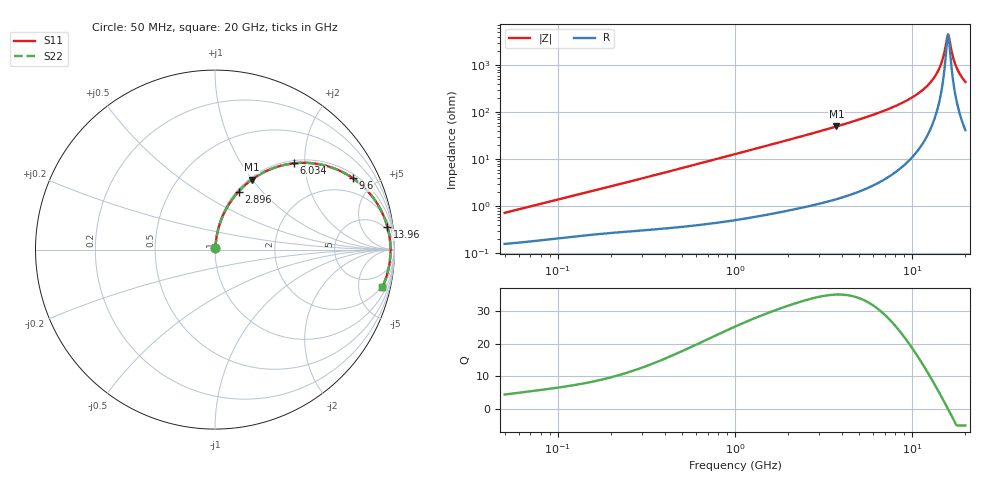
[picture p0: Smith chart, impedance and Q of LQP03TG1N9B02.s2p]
!Murata Part Number: LQP03TG1N9B02
!These Parameters are Measured in Series Mode Connection
!  o--[Z]--o
!Port1  Port2
!  o-------o
!Freq. Start=50[MHz] Stop=20[GHz], 401[Steps]
# Hz S RI R 50
!Freq.(Hz) S11(Real) S11(Imag) S21(Real) S21(Imag) S12(Real) S12(Imag) S22(Real) S22(Imag)
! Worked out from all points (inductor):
!   401 points, 50 MHz to 20 GHz, reference 50 ohm
!   read as one part in series: L = 2.23 nH near 51.52 MHz
!   highest Q = 35.1 at 3.736 GHz (marker M1), where L = 2.11 nH
!   self-resonance near 15.74 GHz
!   S11 on the Smith chart (normalised r, x): 50 MHz: 1.00, +0.01; 2.896 GHz: 1.02, +0.75; 6.034 GHz: 1.06, +1.76; 9.6 GHz: 1.19, +3.74; 13.96 GHz: 3, +14; 20 GHz: 1.83, -8.72
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5e7  0.00163 0.00705  0.9984 -0.00705  0.9984 -0.00705  0.00163 0.00705
1.364002e8  0.0027 0.0183  0.9973 -0.0183  0.9973 -0.0183  0.0027 0.0183
3.721004e8  0.00558 0.0479  0.9944 -0.0479  0.9944 -0.0479  0.00558 0.0479
1e9  0.0209 0.1247  0.9791 -0.1247  0.9791 -0.1247  0.0209 0.1247
2.728004e9  0.1182 0.3084  0.8818 -0.3084  0.8818 -0.3084  0.1182 0.3084
2.896447e9  0.1313 0.3234  0.8687 -0.3234  0.8687 -0.3234  0.1313 0.3234
3.736399e9  0.2039 0.3889  0.7961 -0.3889  0.7961 -0.3889  0.2039 0.3889
6.034176e9  0.4382 0.4807  0.5618 -0.4807  0.5618 -0.4807  0.4382 0.4807
7.442007e9  0.5819 0.4754  0.4181 -0.4754  0.4181 -0.4754  0.5819 0.4754
9.600142e9  0.7673 0.3984  0.2327 -0.3984  0.2327 -0.3984  0.7673 0.3984
1.201863e10  0.9042 0.2554  0.0958 -0.2554  0.0958 -0.2554  0.9042 0.2554
1.314879e10  0.9423 0.1809  0.0577 -0.1809  0.0577 -0.1809  0.9423 0.1809
1.396067e10  0.9605 0.1273  0.0395 -0.1273  0.0395 -0.1273  0.9605 0.1273
1.482269e10  0.9725 0.0715  0.0275 -0.0715  0.0275 -0.0715  0.9725 0.0715
1.573793e10  0.9778 0.0143  0.0222 -0.0143  0.0222 -0.0143  0.9778 0.0143
1.597544e10  0.9781 -2.71e-05  0.0219 2.71e-05  0.0219 2.71e-05  0.9781 -2.71e-05
1.621653e10  0.978 -0.0144  0.022 0.0144  0.022 0.0144  0.978 -0.0144
1.646126e10  0.9774 -0.0288  0.0226 0.0288  0.0226 0.0288  0.9774 -0.0288
1.721783e10  0.9731 -0.0716  0.0269 0.0716  0.0269 0.0716  0.9731 -0.0716
1.774144e10  0.9682 -0.0999  0.0318 0.0999  0.0318 0.0999  0.9682 -0.0999
1.88369e10  0.9535 -0.155  0.0465 0.155  0.0465 0.155  0.9535 -0.155
2e10  0.9327 -0.2076  0.0673 0.2076  0.0673 0.2076  0.9327 -0.2076
